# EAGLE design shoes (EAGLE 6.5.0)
AUTHOR: Brad Campbell; REV: A; TITLE: Shoes!
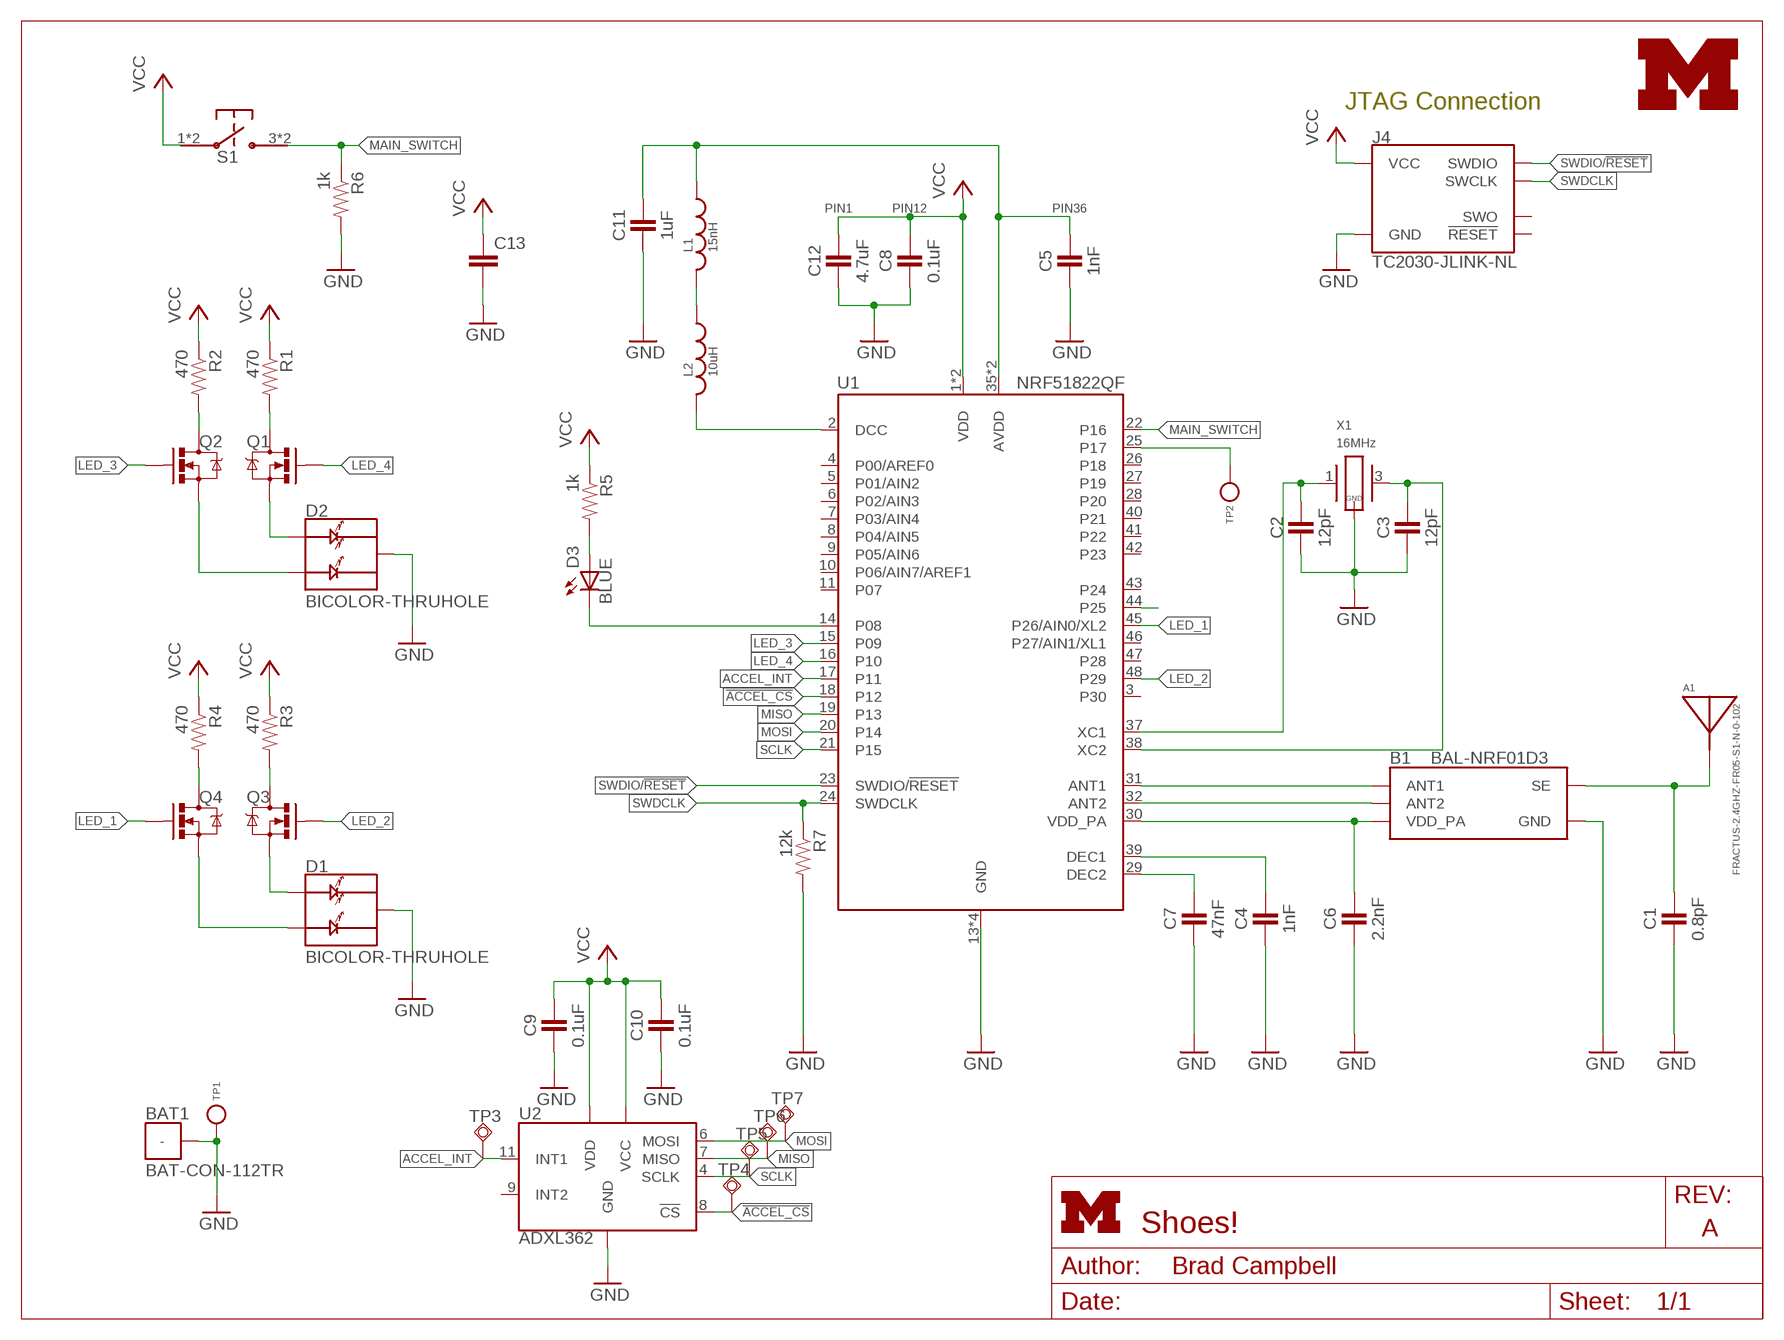
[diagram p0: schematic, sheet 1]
FRAME1 (LETTER_L): HEIGHT: 8.5in; WIDTH: 11in

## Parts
A1  FRACTUS-2.4GHZ-FR05-S1-N-0-102  [FRACTUS-ANTENNA-FR05-S1-N-0-102]
B1  BAL-NRF01D3  [BAL-NRF01D3]
BAT1  BAT-CON-112TR  [BAT-CON-112TR]
C1  0.8pF  CAPACITOR  [0402_CAP]
C2  12pF  CAPACITOR  [0402_CAP]
C3  12pF  CAPACITOR  [0402_CAP]
C4  1nF  CAPACITOR  [0402_CAP]
C5  1nF  CAPACITOR  [0402_CAP]
C6  2.2nF  CAPACITOR  [0402_CAP]
C7  47nF  CAPACITOR  [0402_CAP]
C8  0.1uF  CAPACITOR  [0402_CAP]
C9  0.1uF  CAPACITOR  [0402_CAP]
C10  0.1uF  CAPACITOR  [0402_CAP]
C11  1uF  CAPACITOR  [0402_CAP]
C12  4.7uF  CAPACITOR  [0402_CAP]
C13  CAP0805  [0805]
D1  BICOLOR-THRUHOLE  [3AXIS-0.1IN]
D2  BICOLOR-THRUHOLE  [3AXIS-0.1IN]
D3  BLUE  LED0603  [LED-0603]
J4  TC2030-JLINK-NL  [TC2030-IDC-NL]
L1  15nH  INDUCTOR0402  [0402_CAP]
L2  10uH  INDUCTOR0603  [0603_CAP]
LOGO3  UMICH_SOLID_TINY  [UMICH_SOLID_50MIL]
Q1  MOSFET-NCHANNELXFDN-3  [XFDFN-3]
Q2  MOSFET-NCHANNELXFDN-3  [XFDFN-3]
Q3  MOSFET-NCHANNELXFDN-3  [XFDFN-3]
Q4  MOSFET-NCHANNELXFDN-3  [XFDFN-3]
R1  470  RESISTOR  [0402_RES]
R2  470  RESISTOR  [0402_RES]
R3  470  RESISTOR  [0402_RES]
R4  470  RESISTOR  [0402_RES]
R5  1k  RESISTOR  [0402_RES]
R6  1k  RESISTOR  [0402_RES]
R7  12k  RESISTOR  [0402_RES]
S1  TL3315NF100Q  [TL3315NF100Q]
TP1  TEST_POINT_0.020IN  [TESTPOINT_0.020IN]
TP2  TEST_POINT_0.020IN  [TESTPOINT_0.020IN]
TP3  TPSQTP06SQ  [TP06SQ]
TP4  TPSQTP06SQ  [TP06SQ]
TP5  TPSQTP06SQ  [TP06SQ]
TP6  TPSQTP06SQ  [TP06SQ]
TP7  TPSQTP06SQ  [TP06SQ]
U1  NRF51822QF  [QFN-48-6MM]
U2  ADXL362  [TFLGA-16/3.3MMX3.1MM]
X1  16MHz  TXC-8Y  [TXC-8Y]

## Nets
!ACCEL_CS: TP4.TP U1.18(P12) U2.8(!CS)
ACCEL_INT: TP3.TP U1.17(P11) U2.11(INT1)
AVDD: C5.1 C11.1 L1.1 U1.35(AVDD) U1.36(AVDD)
DCC: L2.2 U1.2(DCC)
GND: B1.GND BAT1.PAD(-) C1.2 C2.2 C3.2 C4.2 C5.2 C6.2 C7.2 C8.2 C9.2 C10.2 C11.2 C12.2 C13.2 D1.M(C) D2.M(C) J4.5(GND) R6.2 R7.2 TP1.TESTPOINT U1.13(GND) U1.33(GND) U1.34(GND) U1.GND U2.12(GND) U2.13(GND) U2.16(GND) X1.2(GND) X1.4(GND)
LED_1: Q4.G U1.45(P26/AIN0/XL2)
LED_2: Q3.G U1.48(P29)
LED_3: Q2.G U1.15(P09)
LED_4: Q1.G U1.16(P10)
MAIN_SWITCH: R6.1 S1.3 S1.4 U1.22(P16)
MISO: TP6.TP U1.19(P13) U2.7(MISO)
MOSI: TP7.TP U1.20(P14) U2.6(MOSI)
N$1: TP2.TESTPOINT U1.25(P17)
N$4: D2.1(A1) Q1.S
N$5: B1.ANT1 U1.31(ANT1)
N$6: B1.ANT2 U1.32(ANT2)
N$7: D3.C U1.14(P08)
N$8: D2.2(A2) Q2.S
N$9: Q2.D R2.2
N$10: Q1.D R1.2
N$11: A1.1(ANTENNA) B1.SE C1.1
N$12: D1.1(A1) Q3.S
N$13: D1.2(A2) Q4.S
N$14: L1.2 L2.1
N$15: Q4.D R4.2
N$16: C2.1 U1.37(XC1) X1.1
N$17: C3.1 U1.38(XC2) X1.3
N$18: C4.1 U1.39(DEC1)
N$19: C7.1 U1.29(DEC2)
N$20: Q3.D R3.2
N$23: D3.A R5.2
P25: U1.44(P25)
SCLK: TP5.TP U1.21(P15) U2.4(SCLK)
SWDCLK: J4.4(SWCLK) R7.1 U1.24(SWDCLK)
SWDIO/!RESET: J4.2(SWDIO) U1.23(SWDIO/!RESET)
VCC: C8.1 C9.1 C10.1 C12.1 C13.1 J4.1(VCC) R1.1 R2.1 R3.1 R4.1 R5.1 S1.1 S1.2 U1.1(VDD) U1.12(VDD) U2.1(VDD) U2.14(VCC)
VDD_PA: B1.VCC(VDD_PA) C6.1 U1.30(VDD_PA)
Unconnected: J4.3(!RESET) J4.6(SWO) U1.3(P30) U1.4(P00/AREF0) U1.5(P01/AIN2) U1.6(P02/AIN3) U1.7(P03/AIN4) U1.8(P04/AIN5) U1.9(P05/AIN6) U1.10(P06/AIN7/AREF1) U1.11(P07) U1.26(P18) U1.27(P19) U1.28(P20) U1.40(P21) U1.41(P22) U1.42(P23) U1.43(P24) U1.46(P27/AIN1/XL1) U1.47(P28) U2.9(INT2)

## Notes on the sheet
- JTAG Connection
- PIN1 | PIN12 | PIN36

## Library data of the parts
A1 = chips:FRACTUS-2.4GHZ-FR05-S1-N-0-102: Fractus Compact Reach XtendTM chip antenna is engineered specifically for Bluetooth,; RICHARDSON_RFPD: FR05-S1-N-0102B
B1 = chips:BAL-NRF01D3: 50 ohm nominal input / conjugate match balun to nRF51422-QFAA, nRF24LE1, nRF51822-QFAA/AB, with integrated harmonic filter; DIGIKEY: 497-13637-1-ND; MOUSER: 511-BAL-NRF01D3
BAT1 = batteries:BAT-CON-112TR; DIGIKEY: 36-112CT-ND
C1 = passives:CAPACITOR: 0402 Capacitor; DIGIKEY: 490-6269-1-ND
C2 C3 = passives:CAPACITOR: 0402 Capacitor; DIGIKEY: 490-6197-1-ND
C4 C5 = passives:CAPACITOR: 0402 Capacitor; DIGIKEY: 490-1303-1-ND
C6 = passives:CAPACITOR: 0402 Capacitor; DIGIKEY: 490-5419-1-ND
C7 = passives:CAPACITOR: 0402 Capacitor; DIGIKEY: 445-1264-1-ND
C8-C10 = passives:CAPACITOR: 0402 Capacitor; DIGIKEY: 445-4952-1-ND
C11 = passives:CAPACITOR: 0402 Capacitor; DIGIKEY: 1276-1513-1-ND
C12 = passives:CAPACITOR: 0402 Capacitor; DIGIKEY: 445-5947-1-ND
C13 = SparkFun-Capacitors:CAP: Capacitor
D1 D2 = leds:BICOLOR-THRUHOLE: 3 axis thru-hold LED
D3 = SparkFun-LED:LED: LEDs
J4 = connector:TC2030-JLINK
L1 = passives:INDUCTOR; DIGIKEY: 587-1521-1-ND
L2 = passives:INDUCTOR; DIGIKEY: 490-4025-1-ND
LOGO3 = logos:UMICH_SOLID
Q1-Q4 = fets:MOSFET-NCHANNEL: Generic NMOS footprint; DIGIKEY: DMN2400UFB4-7DICT-ND
R1-R4 = passives:RESISTOR: Resistor; DIGIKEY: RHM470CDCT-ND
R5 R6 = passives:RESISTOR: Resistor; DIGIKEY: RHM1.0KCECT-ND
R7 = passives:RESISTOR: Resistor; DIGIKEY: RHM12.0KCDCT-ND
S1 = switches:TL3315NF100Q: SWITCH TACTILE SPST-NO 0.05A 15V; DIGIKEY: EG4620CT-ND
TP1 TP2 = headers:TEST_POINT_0.020IN
TP3-TP7 = testpad:TPSQ: Test pad
U1 = chips:NRF51822: Multiprotocol Bluetooth® 4.0 low energy/2.4 GHz RF SoC; DIGIKEY: 1490-1032-1-ND; MOUSER: 949-NRF51822-QFAB-R7
U2 = chips:ADXL362: IC ACCEL DIG LO PWR 3AX 16LGA; DIGIKEY: ADXL362BCCZ-RL7CT-ND; MOUSER: 584-ADXL362BCCZ-R7; NEWARK: 47W0478
X1 = crystals:TXC-8Y: 2mmx1.6mm SMD Crystal; DIGIKEY: 887-2003-1-ND

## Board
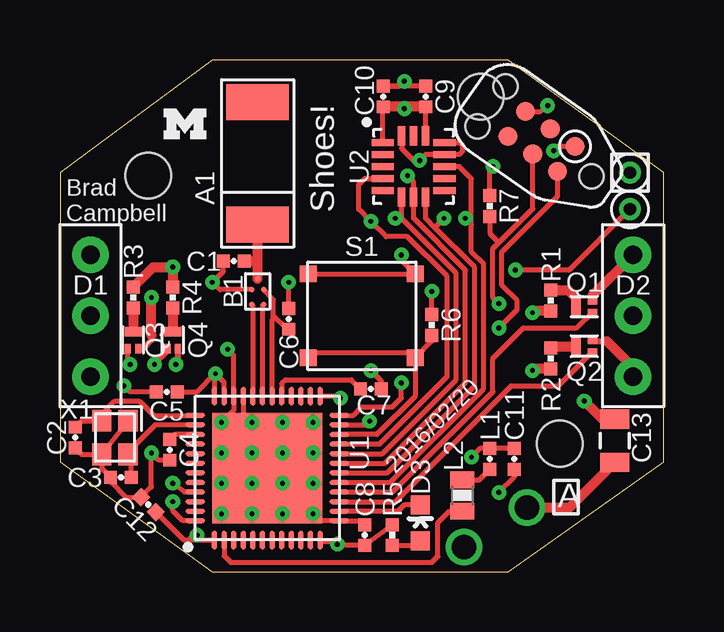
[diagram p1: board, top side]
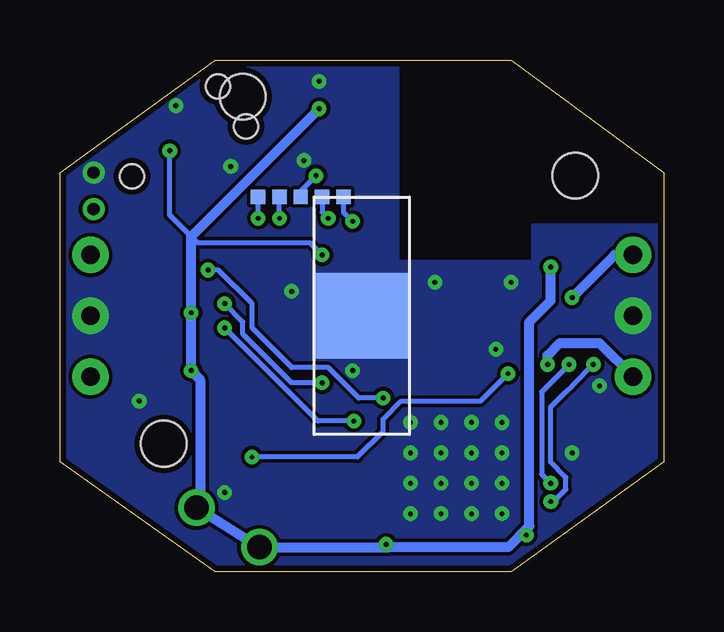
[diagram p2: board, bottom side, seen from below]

Size 25.15 x 21.34 mm. Coordinates in mm from the lower left corner, seen from the top.
Outline: 0,4.57 6.35,0 18.67,0 25.15,4.57 25.15,16.64 18.67,21.34 6.35,21.34 0,16.64 0,4.57
Copper layers (1*16): Top 0.0178mm / dielectric 59mil / Bottom 0.0178mm
Design rules "sunstone-2lyr_v1.0.0.3 *": minimum track width 6mil, minimum drill 8mil, track to track 6mil, track to pad 6mil, pad to pad 6mil, via to via 6mil, smd to smd 6mil, copper to edge 10mil, drill to drill 16mil, minimum pad ring 8mil, minimum via ring 8mil, stop-mask expansion 3mil, vias tented up to drill 50mil, thermal gap 10mil
Holes 1.91 mm at 3.68,16.51 17.53,19.81 20.83,5.33

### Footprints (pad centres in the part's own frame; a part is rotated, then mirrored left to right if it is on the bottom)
FRACTUS-ANTENNA-FR05-S1-N-0-102 = smd 1.5 x 2.6: 1 -2.55,0; 2 2.55,0
BAL-NRF01D3 = smd 0.22 x 0.22: ANT1 -0.537,-0.25; ANT2 -0.537,0.25; GND 0.069,0.25; SE 0.537,0; VCC 0.069,-0.25
BAT-CON-112TR = smd 3.962 x 3.556: PAD 0,0
0402_CAP = smd 0.536 x 0.546: 1 -0.433,0; 2 0.433,0
0805 = smd 0.8 x 1.2: 1 -0.9,0; 2 0.9,0
3AXIS-0.1IN = drill 0.762 pad 1.524: 1 -2.54,0; 2 2.54,0; M 0,0
LED-0603 = smd 0.8 x 0.8: A 0,-0.75; C 0,0.75
TC2030-IDC-NL = smd 0.787 x 0.787: 1 -1.27,-0.635; 2 -1.27,0.635; 3 0,-0.635; 4 0,0.635; 5 1.27,-0.635; 6 1.27,0.635 | hole 1.016: -2.54,0; 2.54,1.016; 2.54,-1.016
0603_CAP = smd 0.7 x 1: 1 -0.65,0; 2 0.65,0
XFDFN-3 = smd 0.4 x 0.7: D 0.35,0 | smd 0.4 x 0.25: G -0.35,0.215; S -0.35,-0.215
0402_RES = smd 0.536 x 0.546: 1 -0.433,0; 2 0.433,0
TL3315NF100Q = smd 0.7 x 0.7: 1 -2.225,1.75; 2 2.225,1.75; 3 -2.225,-1.75; 4 2.225,-1.75
TESTPOINT_0.020IN = drill 0.508: TESTPOINT 0,0
TP06SQ = smd 0.6 x 0.6: TP 0,0
QFN-48-6MM = smd 0.8 x 0.203: 1 -3,2.2; 2 -3,1.8; 3 -3,1.4; 4 -3,1; 5 -3,0.6; 6 -3,0.2; 7 -3,-0.2; 8 -3,-0.6; 9 -3,-1; 10 -3,-1.4; 11 -3,-1.8; 12 -3,-2.2; 25 3,-2.2; 26 3,-1.8; 27 3,-1.4; 28 3,-1; 29 3,-0.6; 30 3,-0.2; 31 3,0.2; 32 3,0.6; 33 3,1; 34 3,1.4; 35 3,1.8; 36 3,2.2 | smd 0.203 x 0.8: 13 -2.2,-3; 14 -1.8,-3; 15 -1.4,-3; 16 -1,-3; 17 -0.6,-3; 18 -0.2,-3; 19 0.2,-3; 20 0.6,-3; 21 1,-3; 22 1.4,-3; 23 1.8,-3; 24 2.2,-3; 37 2.2,3; 38 1.8,3; 39 1.4,3; 40 1,3; 41 0.6,3; 42 0.2,3; 43 -0.2,3; 44 -0.6,3; 45 -1,3; 46 -1.4,3; 47 -1.8,3; 48 -2.2,3 | smd 4.6 x 4.6: GND 0,0
TFLGA-16/3.3MMX3.1MM = smd 0.925 x 0.3: 1 -1.288,1; 2 -1.288,0.5; 3 -1.288,0; 4 -1.288,-0.5; 5 -1.288,-1; 9 1.288,-1; 10 1.288,-0.5; 11 1.288,0; 12 1.288,0.5; 13 1.288,1 | smd 0.3 x 0.8: 6 -0.5,-1.275; 7 0,-1.275; 8 0.5,-1.275; 14 0.5,1.275; 15 0,1.275; 16 -0.5,1.275
TXC-8Y = smd 0.9 x 0.8: 1 -0.7,-0.55; 2 0.7,-0.55; 3 0.7,0.55; 4 -0.7,0.55

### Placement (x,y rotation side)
A1  8.23,17.02 90 top
B1  8.23,11.68 90 top
BAT1  12.57,10.67 0 bottom
C1  7.24,12.95 180 top
C2  0.63,5.59 270 top
C3  2.54,3.94 180 top
C4  4.57,5.08 270 top
C5  4.45,7.49 180 top
C6  9.53,10.54 90 top
C7  12.95,7.62 0 top
C8  12.7,1.52 90 top
C9  15.24,19.81 90 top
C10  13.46,19.81 90 top
C11  18.92,4.7 270 top
C12  3.68,2.79 135 top
C13  23.11,5.46 90 top
D1  1.27,10.67 270 top
D2  23.88,10.67 270 top
D3  15.01,2.03 0 top
J4  20.06,17.94 145 top
L1  17.91,4.7 270 top
L2  16.76,3.17 270 top
LOGO3  5.21,18.67 0 top
Q1  21.84,11.05 180 top
Q2  21.84,9.4 180 top
Q3  3.05,9.65 90 top
Q4  4.7,9.65 90 top
R1  20.45,11.3 90 top
R2  20.45,8.89 90 top
R3  3.05,11.43 270 top
R4  4.7,11.43 270 top
R5  13.84,1.52 270 top
R6  15.49,10.29 90 top
R7  17.91,15.24 90 top
S1  12.57,10.67 0 top
TP1  23.75,16.64 0 top
TP2  23.75,15.11 0 top
TP3  16.89,15.62 0 bottom
TP4  16,15.62 0 bottom
TP5  13.34,15.62 0 bottom
TP6  15.11,15.62 0 bottom
TP7  14.22,15.62 0 bottom
U1  8.64,4.32 90 top
U2  14.73,16.89 0 top
X1  2.29,5.59 270 top

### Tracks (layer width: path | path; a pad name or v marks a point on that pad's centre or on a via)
!ACCEL_CS  (via drill 0.2)
  Top 0.203: U1.18 13.64,4.12 17.27,7.75 17.27,12.7 15.62,14.35 | 15.23,15.5 U2.8 15.23,14.74 15.62,14.35 | 15.62,14.35 v16,14.73
  Bottom 0.203: v16,14.73 TP4.TP
ACCEL_INT  (via drill 0.2)
  Top 0.203: U1.17 13.75,3.72 17.65,7.62 17.65,12.83 17.14,13.33 17.14,14.48 | 17.14,14.48 17.14,16.38 16.64,16.89 U2.11 | v16.89,14.73 17.14,14.48
  Bottom 0.203: v16.89,14.73 TP3.TP
AVDD  (via drill 0.2)
  Top 0.203: C11.1 L1.1 17.5,5.13 v17.14,4.77 | 6.44,7.41 U1.36 | U1.35 6.84,7.9 v6.48,8.25 | 6.44,7.71 U1.36 | C5.1 5.72,7.49 v6.48,8.25 | v6.48,8.25 6.44,8.21 U1.36
  Bottom 0.203: v6.48,8.25 7.62,7.11 10.92,7.11 11.68,6.35 11.68,5.84 12.75,4.77 v17.14,4.77
DCC
  Top 0.203: U1.2 6.84,0.66 7.11,0.38 15.49,0.38 15.75,0.63 15.75,2.03 16.24,2.52 L2.2
GND  (via drill 0.2)
  Top 0.203: C2.2 0.9,4.89 X1.2 | X1.2 1.74,4.31 C3.2 2.11,3.73 2.74,3.1 C12.2 3.81,3.53 v3.81,4.95 4.12,4.65 C4.2 | X1.2 X1.4 | v10.54,2.41 10.84,2.12 U1.13 12.54,2.12 C8.2 | v6.73,6.22 7.24,6.73 U1.34 7.24,9.02 v6.99,9.27 | U1.33 7.64,6.59 v8,6.22 | U1.GND v9.27,4.95 | C5.2 2.92,7.49 v2.67,7.75 | J4.5 20.01,19.18 v20.32,19.43 | U2.16 14.23,17.64 14.73,17.14 v14.99,17.14 15.23,17.39 U2.12 16.63,17.39 16.76,17.53 16.76,17.78 16.65,17.89 U2.13 | C9.2 C10.2 14.15,20.24 v14.35,20.45 | C11.2 18.92,3.94 v18.29,3.3 | C7.2 13.39,7.95 v12.95,8.38 | R7.2 17.91,16.76 v18.03,16.89 | R6.2 v15.49,11.68 | C1.2 6.81,12.52 v6.35,12.06 6.66,11.75 B1.GND | C6.2 v9.53,12.06
  Top 0.406: 23.12,6.35 C13.2 22.59,6.36 v21.84,7.11
  other vias: 9.27,3.68 8,3.68 6.73,3.68 6.73,2.41 8,2.41 9.27,2.41 10.54,3.68 6.73,4.95 8,4.95 10.54,4.95 9.27,6.22 10.54,6.22
  pour Bottom (no thermals): 0,14.48 5.46,14.48 5.46,12.95 11.05,12.95 11.05,21.34 18.67,21.34 25.15,16.64 25.15,4.57 18.67,0 6.35,0 0,4.57
LED_1  (via drill 0.2)
  Top 0.203: U1.45 5.19,3.32 v4.7,3.68 | Q4.G 4.48,9.18 v3.94,8.64
  Bottom 0.203: v3.94,8.64 5.08,7.49 5.08,4.06 v4.7,3.68
LED_2  (via drill 0.2)
  Top 0.203: U1.48 5.12,2.12 4.7,2.54 v4.7,2.92 | v2.92,8.64 2.83,8.72 Q3.G
  Bottom 0.203: v2.92,8.64 3.81,7.75 4.06,7.49 4.7,6.86 4.7,4.57 4.06,3.94 4.06,3.43 4.57,2.92 v4.7,2.92
LED_3
  Top 0.203: U1.15 13.97,2.92 18.8,7.75 20.76,7.75 Q2.G
LED_4
  Top 0.203: Q1.G 21.52,10.16 19.3,10.16 18.03,8.89 18.03,7.49 13.86,3.32 U1.16
MAIN_SWITCH
  Top 0.203: S1.4 14.8,7.3 13.21,5.71 U1.22 | S1.3 10.57,9.14 14.57,9.14 S1.4 | S1.4 15.49,9.61 R6.1
MISO  (via drill 0.2)
  Top 0.203: U1.19 13.54,4.52 16.89,7.87 16.89,12.57 14.73,14.73 U2.7 14.73,16.26 v14.48,16.51
  Bottom 0.203: v14.48,16.51 15.11,15.88 TP6.TP
MOSI  (via drill 0.2)
  Top 0.203: U1.20 13.43,4.92 16.51,8 16.51,12.45 14.23,14.72 | 14.23,14.72 U2.6 | 14.23,14.72 v13.98,14.72 v13.97,14.73
  Bottom 0.203: TP7.TP 14.22,14.99 v13.97,14.73
N$1  (via drill 0.2)
  Top 0.203: U1.25 11.61,7.32 v11.68,7.24 | TP2.TESTPOINT 21.21,12.57 v18.97,12.57
  Bottom 0.203: v11.68,7.24 12.7,7.24 13.97,8.51 15.49,8.51 17.14,10.16 17.14,11.18 18.54,12.57 v18.97,12.57
N$4
  Top 0.254: Q1.S 22.19,11.53
  Top 0.406: 22.19,11.53 D2.1
N$5
  Top 0.203: B1.ANT1 8.44,11.1 U1.31
N$6
  Top 0.203: B1.ANT2 8.04,11.09 U1.32
N$7
  Top 0.203: D3.C 14.34,2.78 14.08,2.52 U1.14
N$8
  Top 0.254: Q2.S 22.77,9.61
  Top 0.406: 22.77,9.61 23.88,8.51 D2.2
N$9
  Top 0.406: R2.2 20.52,9.4 Q2.D
N$10
  Top 0.406: R1.2 21.16,11.74 21.49,11.4 Q1.D
N$11
  Top 0.406: B1.SE 8.23,12.95 | 8.23,12.95 A1.1 | C1.1 8.23,12.95
N$12  (via drill 0.2)
  Top 0.254: Q3.S 3.46,9.3 3.81,9.65 3.81,9.85
  Top 0.406: 3.81,9.85 v3.81,11.43
  Bottom 0.406: v3.81,11.43 2.03,13.21 D1.1
N$13  (via drill 0.2)
  Top 0.254: Q4.S 4.91,8.72
  Top 0.406: 4.91,8.72 v4.83,8.64
  Bottom 0.406: v4.83,8.64 4.83,9.02 4.32,9.52 2.67,9.52 D1.2
N$14
  Top 0.203: L2.1 17.47,3.82 L1.2
N$15
  Top 0.406: R4.2 Q4.D
N$16
  Top 0.203: C2.1 0.9,6.29 X1.1 1.74,6.56 2.29,7.11 3.3,7.11 3.9,6.52 U1.37
N$17
  Top 0.203: C3.1 2.97,4.75 X1.3 2.84,4.99 3.96,6.12 U1.38
N$18
  Top 0.203: U1.39 4.78,5.72 C4.1
N$19
  Top 0.203: U1.29 9.24,7.84 9.4,8 12.14,8 C7.1
N$20
  Top 0.406: R3.2 Q3.D
N$23
  Top 0.203: R5.2 14.82,1.09 D3.A
SCLK  (via drill 0.2)
  Top 0.203: U1.21 13.32,5.32 16.13,8.13 16.13,12.32 14.48,13.97 13.59,13.97 v12.95,14.6 12.45,15.11 12.45,16.13 12.71,16.39 U2.4
  Bottom 0.203: TP5.TP 13.34,14.99 v12.95,14.6
SWDCLK  (via drill 0.2)
  Top 0.203: U1.24 12.23,6.52 12.57,6.86 13.84,6.86 14.22,7.24 v14.22,7.87 | R7.1 17.91,14.1 18.29,13.72 | v18.29,11.18 18.03,11.43 18.03,13.47 18.29,13.72 | 18.29,13.72 19.7,15.13 J4.4
  Bottom 0.203: v14.22,7.87 15.49,7.87 17.53,9.91 17.53,10.41 v18.29,11.18
SWDIO/!RESET  (via drill 0.2)
  Top 0.203: U1.23 12.75,6.12 v12.9,6.27 | v18.29,10.16 19.05,10.92 19.05,11.3 18.41,11.94 18.41,13.33 20.74,15.66 J4.2
  Bottom 0.203: v12.9,6.27 14.4,6.27 v18.29,10.16
VCC  (via drill 0.2, 1.02)
  Top 0.203: U1.12 10.88,1.27 11.43,1.27 v11.56,1.14 11.61,1.09 C8.1 R5.1 | 5.33,1.32 5.16,1.32 C12.1 | 5.33,1.32 U1.1 | v5.72,1.52 5.54,1.52 5.33,1.32 | U2.14 15.23,19.37 C9.1 | U2.1 13.45,19.36 C10.1 | S1.1 S1.2 14.22,12.99 v14.22,13.21 | v20.57,17.55 20.76,17.73 J4.1
  Top 0.406: R4.1 v4.7,12.7 3.88,12.7 R3.1 | R2.1 19.76,8.46 v19.69,8.38 | R1.1 19.76,10.87 v19.69,10.79 | C10.1 14.28,19.38 v14.35,19.3 14.43,19.38 C9.1 | C13.1 21.22,2.67 v19.46,2.67
  Bottom 0.203: 5.59,1.9 5.59,1.65 v5.72,1.52 | v20.57,17.55 20.57,14.86 19.69,13.97 19.43,13.72 14.73,13.72 v14.22,13.21
  Bottom 0.406: v4.7,12.7 4.7,11.3 5.59,10.41 5.59,1.9 6.48,1.02 11.43,1.02 | 11.43,1.02 v11.56,1.14 11.68,1.02 | 11.68,1.02 v16.84,1.02 v19.46,2.67 19.3,2.82 19.3,8 v19.69,8.38 v19.69,10.79 19.69,13.97 v14.35,19.3 | 11.68,1.02 11.43,1.02
VDD_PA
  Top 0.203: C6.1 9.4,10.11 9.4,10.16 8.89,10.67 | U1.30 8.84,10.49 8.89,10.54 8.89,10.67 | 8.89,10.67 8.89,11.34 B1.VCC

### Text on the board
tPlace: Brad / Campbell | Shoes! | 2016/02/20 | A

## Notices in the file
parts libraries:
SparkFun-LED: Licensing: CC v3.0 Share-Alike You are welcome to use this library for commercial purposes.
